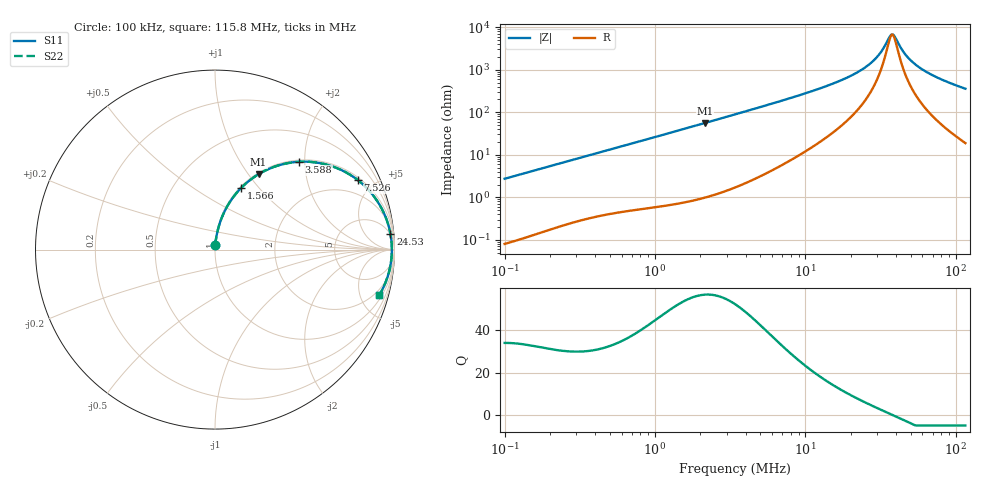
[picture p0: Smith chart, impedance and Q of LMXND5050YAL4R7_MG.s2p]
! LMXND5050YAL4R7_MG  S-PARAMETER MODEL  ( General Type )
! Model Generated by TAIYO YUDEN Corporation (https://www.yuden.co.jp/en/)
! Version 1.0
! TAIYO YUDEN Control No. 191023NI43SB-FBB
! Copyright(c) 2019 TAIYO YUDEN CO.,LTD. All Rights Reserved.
! Product Description (link to TY-COMPAS)
! https://ds.yuden.co.jp/TYCOMPAS/or/detail?pn=LMXND5050YAL4R7NMG&u=M
! Products Name : Inductors
! Characteristics :
!  Inductance : 4.7 uH , SRF(min) : 28 MHz , DC Resistance(max) : 0.0377 Ohm
!  Rated Current : Saturation :3300 mA , Temp Rise : 3100 mA (40 degC)
!  Case Size : 4.9 x 4.9 / 0.193 x 0.193 [mm/inch] , Thickness : 4.1 / 0.161 [mm/inch]
!  (Conditions: Temperature = 25 degC , DC Bias Current/Voltage = 0A / 0V)
! External Node Assignments :
!  1  o---GGG---o  2
! GND o---------o GND
! Frequency Range : 0.1MHz  -  115.823372MHz  [ 402 STEP ]
# MHz S RI R 50
! Freq[MHz].  S11 Real  S11 Imag  S21 Real  S21 Imag  S12 Real  S12 Imag  S22 Real  S22 Imag
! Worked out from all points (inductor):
!   401 points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, 100 kHz to 115.8 MHz, reference 50 ohm
!   read as one part in series: L = 4.33 uH near 103.6 kHz
!   highest Q = 56.8 at 2.152 MHz (marker M1), where L = 4.14 uH
!   self-resonance near 37.46 MHz
!   S11 on the Smith chart (normalised r, x): 100 kHz: 1.00, +0.05; 1.566 MHz: 1.02, +0.81; 3.588 MHz: 1.04, +1.88; 7.526 MHz: 1.13, +4.06; 24.53 MHz: 4, +21; 115.8 MHz: 1.38, -7.13
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0.1  0.00155 0.0272  0.9985 -0.0272  0.9985 -0.0272  0.00155 0.0272
0.325976  0.0103 0.0858  0.9897 -0.0858  0.9897 -0.0858  0.0103 0.0858
1.062605  0.076 0.2543  0.924 -0.2543  0.924 -0.2543  0.076 0.2543
1.56632  0.147 0.3449  0.853 -0.3449  0.853 -0.3449  0.147 0.3449
2.15155  0.2426 0.4199  0.7574 -0.4199  0.7574 -0.4199  0.2426 0.4199
3.463838  0.4514 0.4881  0.5486 -0.4881  0.5486 -0.4881  0.4514 0.4881
3.588199  0.4688 0.4894  0.5312 -0.4894  0.5312 -0.4894  0.4688 0.4894
5.01657  0.6334 0.4702  0.3666 -0.4702  0.3666 -0.4702  0.6334 0.4702
7.52619  0.7969 0.3863  0.2031 -0.3863  0.2031 -0.3863  0.7969 0.3863
11.09389  0.8969 0.2809  0.1031 -0.2809  0.1031 -0.2809  0.8969 0.2809
17.54812  0.9576 0.1628  0.0424 -0.1628  0.0424 -0.1628  0.9576 0.1628
24.53359  0.9775 0.0877  0.0225 -0.0877  0.0225 -0.0877  0.9775 0.0877
30.31621  0.9835 0.044  0.0165 -0.044  0.0165 -0.044  0.9835 0.044
32.53216  0.9845 0.0298  0.0155 -0.0298  0.0155 -0.0298  0.9845 0.0298
36.16345  0.9854 0.00877  0.0146 -0.00877  0.0146 -0.00877  0.9854 0.00877
37.46182  0.9855 0.00177  0.0145 -0.00177  0.0145 -0.00177  0.9855 0.00177
38.8068  0.9854 -0.00523  0.0146 0.00523  0.0146 0.00523  0.9854 -0.00523
47.11532  0.9835 -0.044  0.0165 0.044  0.0165 0.044  0.9835 -0.044
52.37441  0.9811 -0.0656  0.0189 0.0656  0.0189 0.0656  0.9811 -0.0656
59.25644  0.9769 -0.0914  0.0231 0.0914  0.0231 0.0914  0.9769 -0.0914
79.97365  0.9593 -0.1586  0.0407 0.1586  0.0407 0.1586  0.9593 -0.1586
115.8234  0.9159 -0.2524  0.0841 0.2524  0.0841 0.2524  0.9159 -0.2524
